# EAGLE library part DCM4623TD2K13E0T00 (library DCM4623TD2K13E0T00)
Isolated DC/DC Converters 4623 DCM 270Vin 12V 500W Source: Datasheet
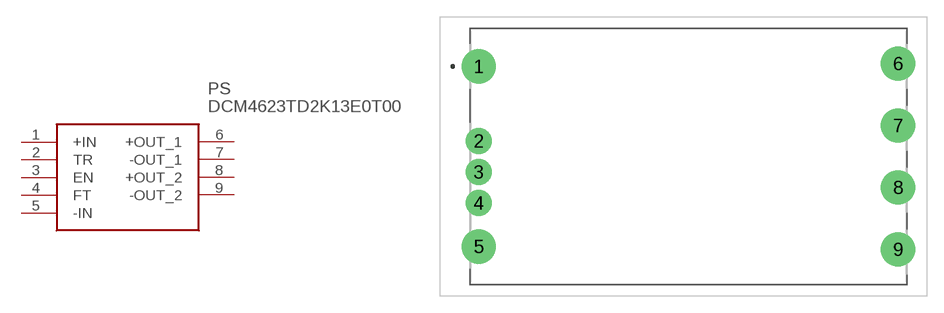
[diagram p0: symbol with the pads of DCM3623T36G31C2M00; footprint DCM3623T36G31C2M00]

Designator prefix PS

## DCM4623TD2K13E0T00 (Description: Isolated DC/DC Converters 4623 DCM 270Vin 12V 500W; Height: mm; Manufacturer_Name: VICOR; Manufacturer_Part_Number: DCM4623TD2K13E0T00; Mouser_Part_Number: 492-DCM4623TD2K13E0T; Mouser_Price-Stock: https://www.mouser.com/Search/Refine.aspx?Keyword=492-DCM4623TD2K13E0T)  [DCM3623T36G31C2M00]
1  +IN
2  TR
3  EN
4  FT
5  -IN
6  +OUT_1
7  -OUT_1
8  +OUT_2
9  -OUT_2

## Footprint DCM3623T36G31C2M00 (pad centres in mm)
DCM MODULE
drill 2.03 pad 3.045: 1 -17.78,8; 5 -17.78,-8; 6 19.42,8.25; 7 19.42,2.75; 8 19.42,-2.75; 9 19.42,-8.25
drill 1.52 pad 2.28: 2 -17.78,1.38; 3 -17.78,-1.38; 4 -17.78,-4.13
